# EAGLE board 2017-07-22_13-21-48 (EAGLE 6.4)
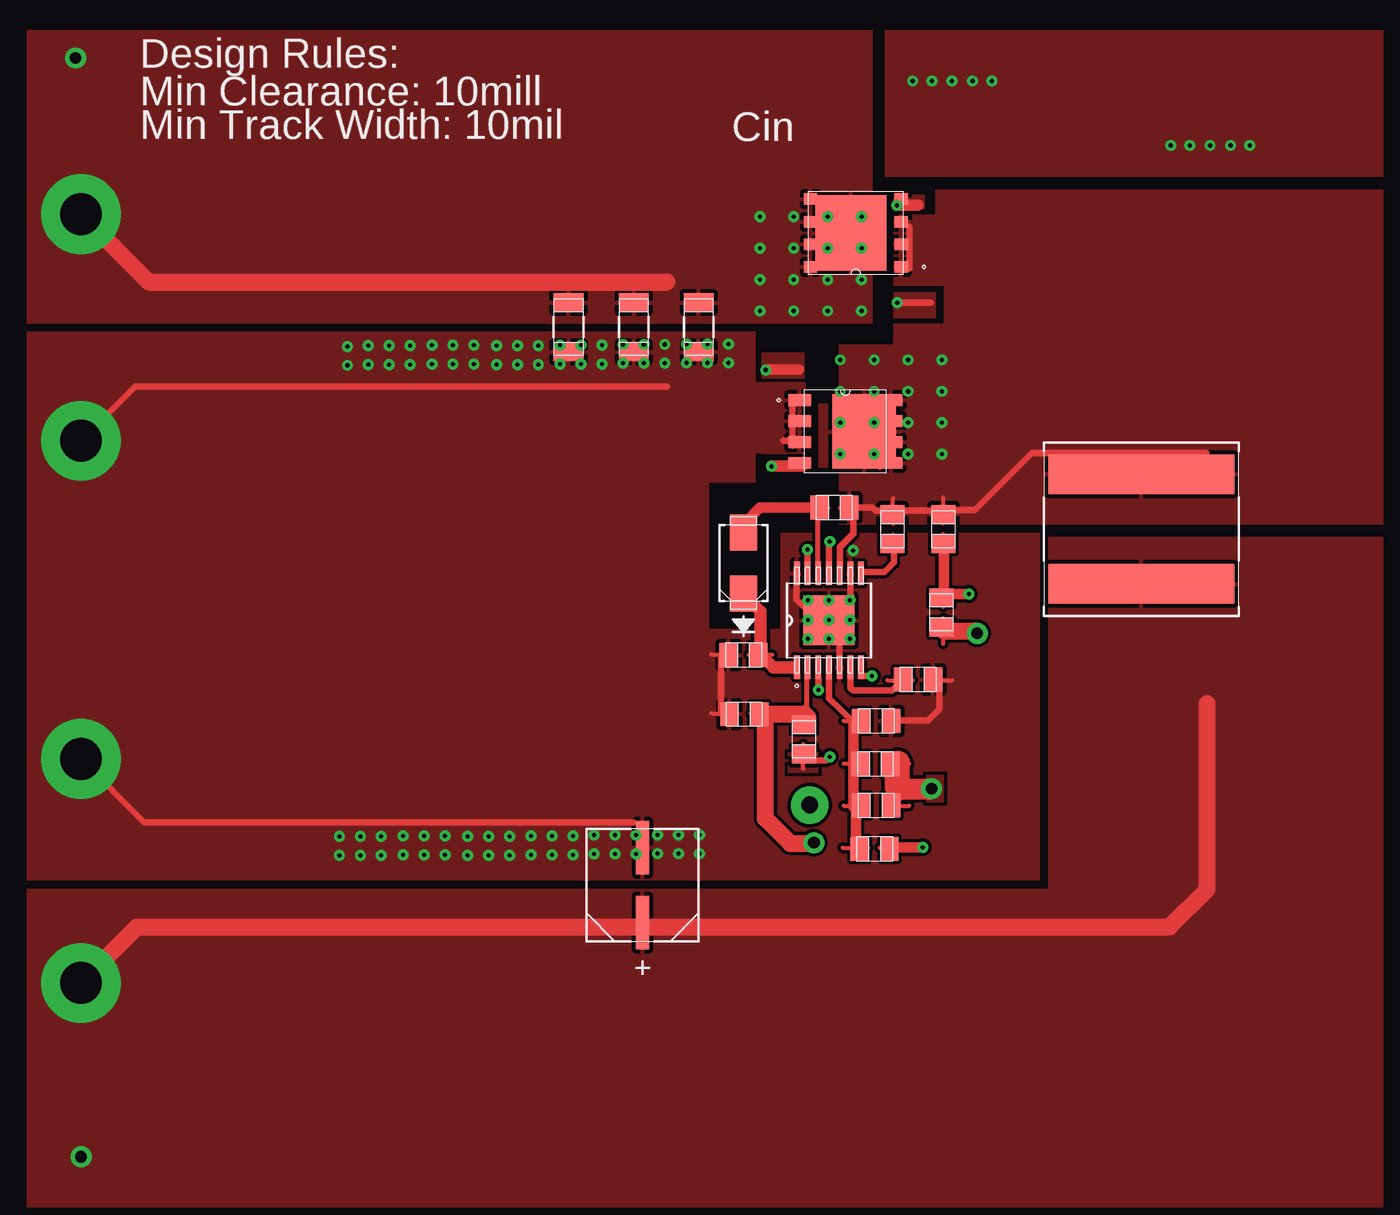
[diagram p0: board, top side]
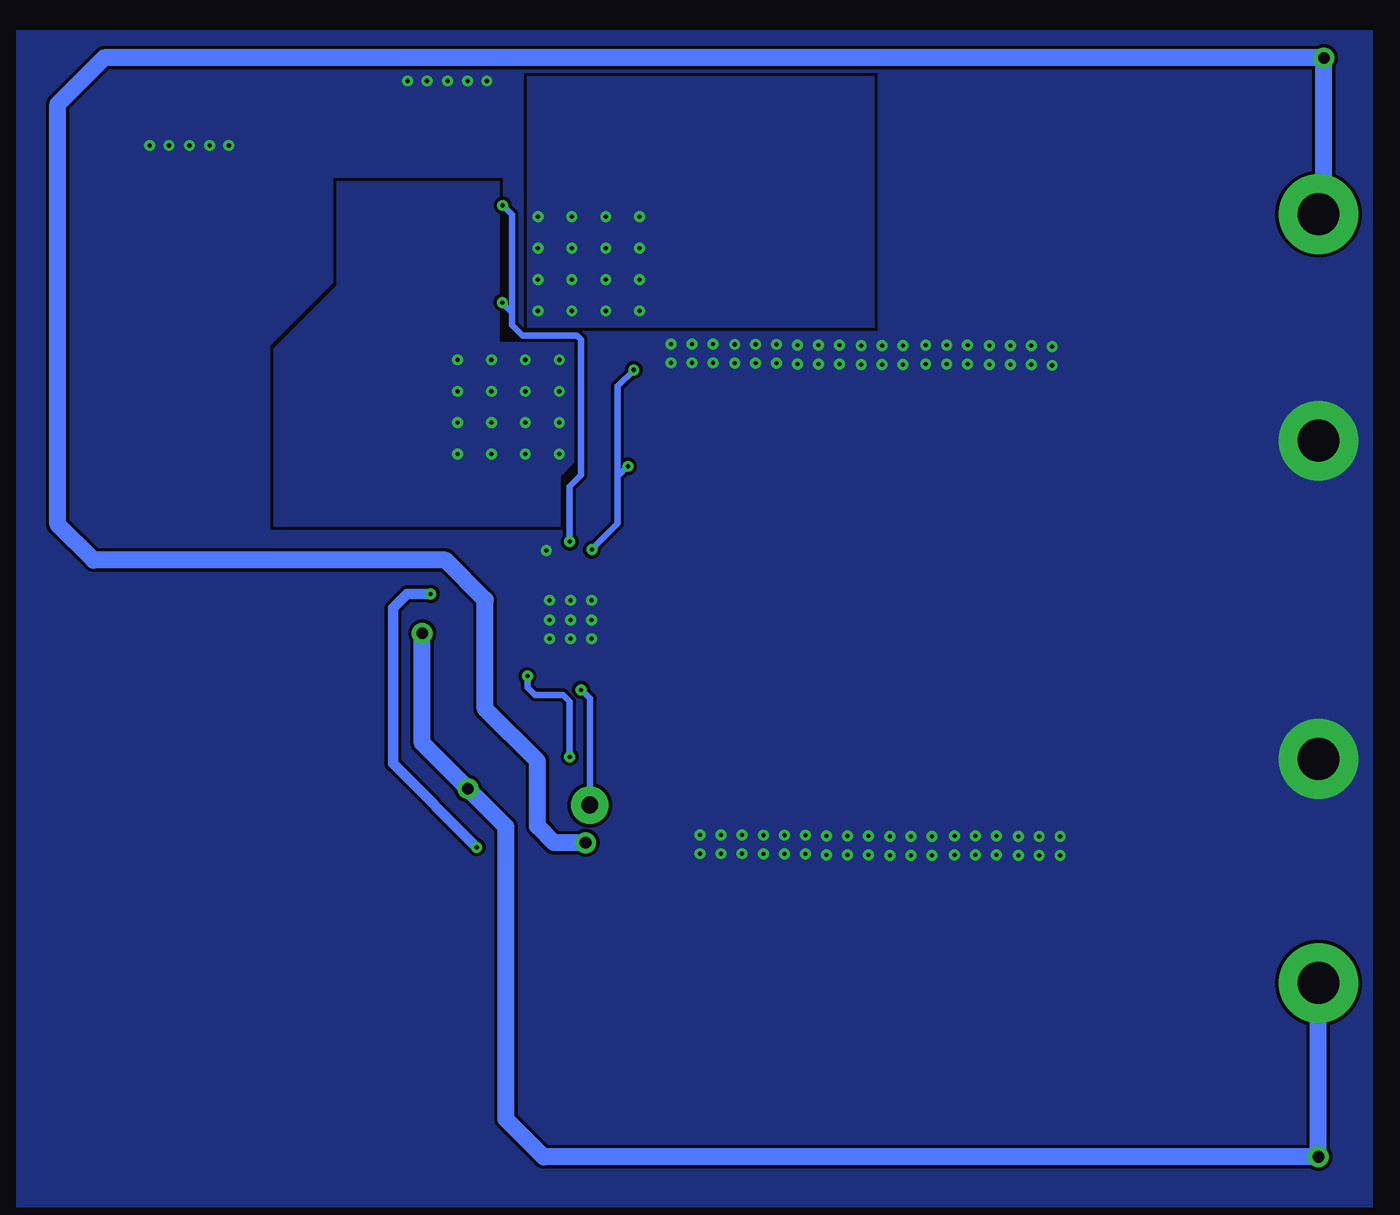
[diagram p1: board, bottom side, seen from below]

No outline drawn. Coordinates in mm, seen from the top.
Copper layers ((1*2)+(15*16)): TOP / INTERNAL1 / layer 15 / BOTTOM

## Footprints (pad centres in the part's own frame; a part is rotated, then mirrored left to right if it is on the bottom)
0805 = smd 1.118 x 1.448: 1 -0.902,0; 2 0.902,0
1206 = smd 1.118 x 1.803: 1 -1.499,0; 2 1.499,0
SM_RADIAL_6.3AMM = smd 3.251 x 0.787: 1 -2.273,0; 2 2.273,0
SMA = smd 2.184 x 1.626: 1 -1.854,0; 2 1.854,0
TP-1502 = drill 0.813 round: 1 0,0
XAL1010 = smd 2.388 x 11.303: 1 -3.327,0; 2 3.327,0
TRANS_NexFET_Q5 = smd 0.8 x 0.7: 1 -2.752,2.055; 2 -2.752,0.685; 3 -2.752,-0.685; 4 -2.752,-2.055; 5 2.752,-2.055; 6 2.752,-0.685; 7 2.752,0.685; 8 2.752,2.055 | smd 4.3 x 4.56: 9 0.3,0
TRANS_NexFET_Q5B = smd 1.37 x 0.71: 1 -2.77,1.905; 2 -2.77,0.635; 3 -2.77,-0.635; 4 -2.77,-1.905; 5 2.77,-1.905; 6 2.77,-0.635; 7 2.77,0.635; 8 2.77,1.905 | smd 3.85 x 4.52: 9 1.16,0
MXA14A = smd 1.422 x 0.356: 1 -2.845,1.95; 2 -2.845,1.3; 3 -2.845,0.65; 4 -2.845,0; 5 -2.845,-0.65; 6 -2.845,-1.3; 7 -2.845,-1.95; 8 2.845,-1.95; 9 2.845,-1.3; 10 2.845,-0.65; 11 2.845,0; 12 2.845,0.65; 13 2.845,1.3; 14 2.845,1.95 | smd 2.997 x 3.099: 15 0,0

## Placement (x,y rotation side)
Cac  [0805]  77.06,47.24 0 top
Cbst  [0805]  74.63,67.94 0 top
Cbyp  [0805]  69.16,55.42 180 top
Cff  [0805]  77.17,49.89 0 top
Cin_1  [1206]  66.4,78.89 270 top
Cin_2  [1206]  62.46,78.89 270 top
Cin_3  [1206]  58.5,78.89 270 top
Cout  [SM_RADIAL_6.3AMM]  62.99,45.06 90 top
Cr  [0805]  81.13,61.59 270 top
Css  [0805]  79.71,57.53 0 top
Cvcc  [0805]  69.11,59 180 top
Dbst  [SMA]  69.11,64.59 90 top
EN  [TP-1502]  73.1,49.89 0 top
GND  [TP-1502]  28.91,71.98 0 top
GND1  [TP-1502]  28.91,52.65 90 top
L1  [XAL1010]  93.24,66.65 270 top
M1  [TRANS_NexFET_Q5]  75.92,84.61 180 top
M2  [TRANS_NexFET_Q5B]  75.29,72.57 0 top
Rfb1  [0805]  77.17,55.02 0 top
Rfb2  [0805]  77.11,52.4 180 top
Rlim  [0805]  78.16,66.65 270 top
Ron  [0805]  72.77,53.9 270 top
Rr  [0805]  81.23,66.65 90 top
U1  [MXA14A]  74.3,61.11 90 top
VIN  [TP-1502]  28.91,85.72 0 top
VOUT  [TP-1502]  28.91,39.07 0 top

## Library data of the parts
Cac = ultra-librarian; RefDes: Cac; Type: C0805C223K5RACTU
Cbst = ultra-librarian; RefDes: Cbst; Type: EMK212B7474KD-T
Cbyp = ultra-librarian; RefDes: Cbyp; Type: 08053C104KAT2A
Cff = ultra-librarian; RefDes: Cff; Type: C0805C102K5RACTU
Cin_1-Cin_3 = ultra-librarian
Cout = ultra-librarian; RefDes: Cout; Type: 6SVPC330M
Cr = ultra-librarian; RefDes: Cr; Type: C0805C223K5RACTU
Css = ultra-librarian; RefDes: Css; Type: CC0805KRX7R9BB153
Cvcc = ultra-librarian; RefDes: Cvcc; Type: EMK212B7105KG-T
Dbst = ultra-librarian; RefDes: Dbst; Type: B350A-13-F
EN = ultra-librarian; RefDes: EN; Type: TP-1502
GND = ultra-librarian; RefDes: GND; Type: TP-1502
GND1 = ultra-librarian; RefDes: GND1; Type: TP-1502
L1 = ultra-librarian; RefDes: L1; Type: XAL1010-472MEB
M1 = ultra-librarian; RefDes: M1; Type: CSD16321Q5
M2 = ultra-librarian; RefDes: M2; Type: CSD18509Q5B
Rfb1 = ultra-librarian; RefDes: Rfb1; Type: ERJ-6ENF1002V
Rfb2 = ultra-librarian; RefDes: Rfb2; Type: ERJ-6ENF7322V
Rlim = ultra-librarian; RefDes: Rlim; Type: C0805C223K5RACTU
Ron = ultra-librarian; RefDes: Ron; Type: ERJ-6ENF2373V
Rr = ultra-librarian; RefDes: Rr; Type: C0805C223K5RACTU
U1 = ultra-librarian; RefDes: U1; Type: LM3150MH/NOPB
VIN = ultra-librarian; RefDes: VIN; Type: TP-1502
VOUT = ultra-librarian; RefDes: VOUT; Type: TP-1502

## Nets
0: Cbyp.2 Cin_1.2 Cin_2.2 Cin_3.2 Cout.2 Css.2 Cvcc.2 GND1.1 GND.1 M2.1 M2.2 M2.3 Rfb1.2 U1.5 U1.9 U1.14 U1.15
1: Css.1 U1.6
2: Cbyp.1 Cin_1.1 Cin_2.1 Cin_3.1 M1.5 M1.6 M1.7 M1.8 M1.9 Ron.1 U1.2 VIN.1
3: Ron.2 U1.7
4: Cff.1 Cout.1 Cr.2 L1.2 Rfb2.1 VOUT.1
5: Cac.1 Cff.2 Rfb1.1 Rfb2.2 U1.4
6: Cbst.2 L1.1 M1.1 M1.2 M1.3 M2.5 M2.6 M2.7 M2.8 M2.9 Rlim.1 Rr.2 U1.10
7: M2.4 U1.13
8: M1.4 U1.11
9: Cbst.1 Dbst.2 U1.12
10: Cvcc.1 Dbst.1 U1.1
11: Rlim.2 U1.8
18: EN.1 U1.3
25: Cac.2 Cr.1 Rr.1

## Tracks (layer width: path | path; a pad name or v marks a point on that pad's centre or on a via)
0  (via drill 0.25 pad 0.51, 2.54 pad 4.83)
  TOP 0.254: 67.16,59.05 68.3,59.05 | 77.67,55.02 79.15,55.02 | 80.21,57.48 81.76,57.48 | 67.16,55.47 68.3,55.47
  TOP 0.381: 81,57.51 81,55.75 80.29,55.04 78.41,55.04 | v28.93,52.7 32.77,48.87 62.43,48.87 | v28.93,72.01 32.21,75.29 64.47,75.29 | 71.53,72.01 71.78,72.01 72.08,71.7 72.08,72.97 72.08,74.24 | 67.74,55.47 67.74,59.05 | 75.59,64.34 75.59,61.75 74.93,61.11 74.93,59.74 | 74.93,58.27 74.93,59.74 | 74.93,59.74 72.31,62.38 72.31,64.21
  other vias: 95.02,89.92 96.19,89.92 97.41,89.92 99.82,89.92 98.65,89.92 83.01,93.83 84.18,93.83 81.76,93.83 80.54,93.83 79.38,93.83 66.45,46.96 65.18,46.96 63.91,46.96 60.05,46.94 61.32,46.94 62.59,46.94 62.59,48.08 61.32,48.08 60.05,48.08 63.91,48.11 65.18,48.11 66.45,48.11 58.78,46.89 57.51,46.89 56.24,46.89 52.37,46.86 53.64,46.86 54.91,46.86 54.91,48.01 53.64,48.01 52.37,48.01 56.24,48.03 57.51,48.03 58.78,48.03 51,46.89 49.73,46.89 48.46,46.89 44.6,46.86 45.87,46.86 47.14,46.86 47.14,48.01 45.87,48.01 44.6,48.01 48.46,48.03 49.73,48.03 51,48.03 45.09,77.72 45.09,76.58 52.76,77.8 51.49,77.8 50.22,77.8 46.35,77.77 47.62,77.77 48.9,77.77 48.9,76.63 47.62,76.63 46.35,76.63 50.22,76.66 51.49,76.66 52.76,76.66 60.53,77.8 59.26,77.8 57.99,77.8 54.13,77.77 55.4,77.77 56.67,77.77 56.67,76.63 55.4,76.63 54.13,76.63 57.99,76.66 59.26,76.66 60.53,76.66 68.2,77.88 66.93,77.88 65.66,77.88 61.8,77.85 63.07,77.85 64.34,77.85 64.34,76.71 63.07,76.71 61.8,76.71 65.66,76.73 66.93,76.73 68.2,76.73 75.56,61.14 74.3,61.14 73.03,61.14 73.03,59.99 74.3,59.99 75.56,59.99 75.56,62.33 74.3,62.33 73.03,62.33 75.77,65.35
  pour TOP (rank 5): 70.21,71.2 70.21,72.77 72.8,72.77 72.8,71.2
  pour TOP (rank 5): 77.7,96.9 77.7,88.01 107.92,88.01 107.92,96.9
  pour TOP (rank 6): 25.63,78.61 69.82,78.61 69.82,75.56 72.87,75.56 72.87,71.25 69.82,71.25 69.82,69.47 67.03,69.47 67.03,60.58 71.35,60.58 71.35,66.42 87.1,66.42 87.1,45.34 25.63,45.34
  pour BOTTOM (rank 6): 25.63,25.53 25.63,96.9 107.92,96.9 107.92,25.53
1
  TOP 0.254: 77.83,57.48 79.38,57.48
  TOP 0.381: U1.6 75.59,57.02 75.79,56.84 78.11,56.84 79.12,57.86
2  (via drill 0.25 pad 0.51, 0.71 pad 1.27, 2.54 pad 4.83)
  TOP 0.254: 72.72,54.36 72.72,55.83 | 69.55,55.45 70.97,55.45
  TOP 0.305: 72.97,58.27 72.97,55.63 72.8,55.45
  TOP 1.016: v28.93,85.75 33.05,81.64 64.47,81.64 | v73.38,47.62 73.33,47.57 71.96,47.57 70.43,49.1 70.43,55.37 70.33,55.37 70.26,55.45 72.8,55.45 73,55.24
  BOTTOM 1.016: 28.93,85.72 28.6,86.06 v28.6,95.22 102.59,95.22 105.39,92.43 105.39,66.93 103.23,64.77 81.89,64.77 79.48,62.36 79.48,55.75 76.3,52.58 76.3,48.64 75.29,47.62 73.46,47.62
  other vias: 70.1,85.6 72.16,85.6 74.22,85.6 76.28,85.6 76.28,83.69 74.22,83.69 72.16,83.69 70.1,83.69 76.28,81.79 74.22,81.79 72.16,81.79 70.1,81.79 76.28,79.88 74.22,79.88 72.16,79.88 70.1,79.88
  pour TOP (rank 2): 73.81,82.4 73.81,86.28 77.62,86.28 77.62,82.4
  pour TOP (rank 3): 25.63,96.9 76.94,96.9 76.94,79.12 25.63,79.12
  pour BOTTOM (rank 5): 55.85,94.11 76.94,94.11 76.94,78.87 55.85,78.87
3  (via drill 0.25 pad 0.51)
  TOP 0.254: 72.72,52.12 72.72,53.59
  TOP 0.381: 76.33,57.73 v76.91,57.73 | 74.32,52.81 74.12,52.6 73.43,52.6
  BOTTOM 0.381: v76.91,57.73 76.91,57.05 76.45,56.59 74.75,56.59 74.35,56.19 v74.35,52.83
  pour TOP: 71.81,51.87 71.81,53.34 73.66,53.34 73.66,51.87
4  (via drill 0.71 pad 1.27, 2.54 pad 4.83)
  TOP 0.254: 77.67,49.86 79.15,49.86 | 77.67,52.43 79.15,52.43 | 81.23,59.69 81.23,61.24
  TOP 1.016: 97.23,56.06 97.23,44.81 94.94,42.52 62.43,42.52 32.33,42.52 v28.93,39.12 | v83.29,60.33 83.13,60.48 81.25,60.48
  TOP 1.27: 78.46,50.9 v80.52,50.9
  TOP 1.524: 78.46,50.9 78.46,52.45
  BOTTOM 1.016: v28.93,39.12 v28.93,28.57 75.92,28.57 78.21,30.86 78.21,48.59 v80.52,50.9 83.29,53.67 v83.29,60.33
  pour TOP (rank 4): 25.63,25.53 25.63,44.83 87.6,44.83 87.6,66.17 107.92,66.17 107.92,25.53
  pour TOP (rank 4): 80.21,51.74 80.21,50.06 81.25,50.06 81.25,51.74
5
  TOP 0.254: 75.18,55.02 76.66,55.02 | 75.18,49.86 76.66,49.86 | 75.18,52.43 76.66,52.43 | 75.13,47.32 76.68,47.32
  TOP 0.381: U1.4 74.3,58.24 74.3,56.39 75.77,54.94
  TOP 0.635: 75.92,47.35 75.92,49.89 | 75.79,49.78 75.77,49.81 75.77,54.94 75.77,55.04
6  (via drill 0.25 pad 0.51)
  TOP 0.254: 74.98,67.92 76.53,67.92 | 78.18,66.98 78.18,68.53 | 81.23,67 81.23,68.56
  TOP 0.381: 77.39,70.43 77.39,71.7 | 79.17,84.99 79.17,83.72 79.17,82.45 | 97.18,71.25 86.59,71.25 83.13,67.79 81.25,67.79 81.23,67.77 78.21,67.77 77.11,67.77 76.94,67.94 75.77,67.94 75.77,66.42 | 75.77,66.42 75.77,66.34 74.95,65.53 74.95,63.86 | 74.98,65.63 75.77,66.42
  other vias: 74.98,71.2 77.04,71.2 79.1,71.2 81.15,71.2 74.98,73.1 77.04,73.1 79.1,73.1 81.15,73.1 74.98,75.01 77.04,75.01 79.1,75.01 81.15,75.01 81.15,76.91 79.1,76.91 77.04,76.91 74.98,76.91
  pour TOP (rank 3): 73.66,70.38 73.66,74.27 77.47,74.27 77.47,70.38
  pour TOP (rank 3): 74.9,66.93 74.9,77.85 78.21,77.85 78.21,79.12 81.25,79.12 81.25,81.41 78.21,81.41 78.21,85.72 80.75,85.72 80.75,87.25 107.92,87.25 107.92,66.93
  pour BOTTOM (rank 4): 78.59,87.76 88.49,87.76 88.49,81.41 92.3,77.6 92.3,66.8 74.9,66.8 74.9,69.85 74.02,70.74 74.02,77.98 78.59,77.98 78.59,86.11
7  (via drill 0.25 pad 0.51)
  TOP 0.381: 73,64.62 v73,65.41
  TOP 0.635: 70.48,76.33 72.49,76.33
  TOP 0.711: v70.81,70.46 72.67,70.46
  BOTTOM 0.381: 71.45,69.85 71.45,75.31 v70.46,76.3 | 71.45,69.85 71.45,66.98 73,65.43 73,65.38 | 71.45,69.85 70.84,70.46 v70.81,70.46
  pour TOP: 70.21,75.77 70.21,77.34 72.8,77.34 72.8,75.77
  pour TOP (rank 2): 71.35,70.13 71.35,70.71 72.85,70.71 72.85,70.13
8  (via drill 0.25 pad 0.51)
  TOP 0.381: v78.44,80.39 80.49,80.39 | 74.3,64.06 74.3,65.86 74.32,65.89
  TOP 0.711: v78.41,86.28 79.7,86.28
  BOTTOM 0.381: 77.88,79.81 78.44,80.37 v78.44,80.39 | v78.41,86.28 77.85,85.72 77.85,79.02 77.22,78.38 73.89,78.38 73.66,78.16 73.66,69.93 74.35,69.24 v74.35,65.89
  pour TOP: 78.21,79.45 78.21,81.03 80.8,81.03 80.8,79.45
  pour TOP (rank 2): 78.21,86.06 78.21,86.94 80.11,86.94 80.11,86.06
9
  TOP 0.254: 69.14,65.81 69.14,67.44 | 72.82,67.92 74.24,67.92
  TOP 0.305: 73.64,64.06 73.64,67.77 73.48,67.94
  TOP 0.635: 73.48,67.94 70.1,67.94 69.19,67.03 69.19,66.45
10
  TOP 0.254: 69.14,61.8 69.14,63.42 | 69.42,59.03 70.84,59.03
  TOP 0.762: 69.16,62.61 70.13,61.65 70.13,59.08 | 70.13,59.03 70.92,58.24 72.19,58.24
11
  TOP 0.254: 78.18,64.75 78.18,66.29
  TOP 0.381: 76.22,64.06 77.67,64.06 78.23,64.62 78.23,65.63
18  (via drill 0.25 pad 0.51, 1.02 pad 2.29)
  TOP 0.381: 73.66,56.92 73.66,57.63
  BOTTOM 0.381: 73.66,56.92 73.1,56.36 73.1,49.78
  other vias: 73.66,56.9 73.13,49.91
25  (via drill 0.25 pad 0.51)
  TOP 0.254: 81.23,64.77 81.23,66.32 | 81.23,61.92 81.23,63.48 | 77.37,47.32 78.92,47.32
  TOP 0.635: 78.16,47.35 v79.98,47.35 | 81.13,62.84 81.25,62.97 81.25,65.56 | 81.25,62.71 v82.78,62.71
  BOTTOM 0.635: v79.98,47.35 85.06,52.43 85.06,61.85 84.2,62.71 v82.78,62.71

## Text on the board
ASSYNOTES: Design Rules: | Min Clearance: 10mill | Min Track Width: 10mil | Cin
